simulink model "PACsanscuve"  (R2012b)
settings: Solver=ode3  StartTime=0.0  StopTime=50  RelTol=1e-3
libraries: simulink x1

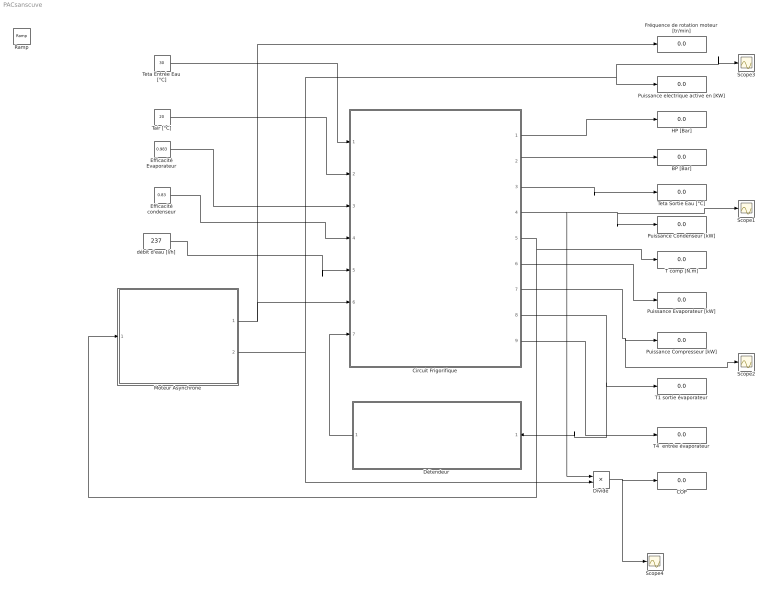
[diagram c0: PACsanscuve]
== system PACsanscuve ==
  BP [Bar] : Display
  COP : Display
  Circuit Frigorifique : Subsystem
  Divide : Product  Inputs=*/
  Détendeur : Subsystem
  Efficacité Evaporateur : Constant  Value=0.983
  Efficacité condenseur : Constant  Value=0.83
  Fréquence de rotation moteur [tr/min] : Display
  HP [Bar] : Display
  Moteur Asynchrone : Subsystem
  Puissance Compresseur [kW] : Display
  Puissance Condenseur [kW] : Display
  Puissance Evaporateur [kW] : Display
  Puissance electrique active en [KW] : Display
  Ramp : simulink/Sources/Ramp  slope=1  start=10  X0=30
  Scope{1..4} (4 alike) : Scope
  T comp [N.m] : Display
  T1 sortie évaporateur : Display
  T4  entrée évaporateur : Display
  Tair [°C] : Constant  Value=20
  Teta Entrée Eau [°C] : Constant  Value=30
  Teta Sortie Eau [°C] : Display
  débit d'eau [l/h] : Constant  Value=237
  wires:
  Efficacité Evaporateur/1 -> Circuit Frigorifique/3(Eff Evapo)
  débit d'eau [l/h]/1 -> Circuit Frigorifique/5(Qv eau [l/h])
  Circuit Frigorifique/1(HP [bar]) -> HP [Bar]/1
  Circuit Frigorifique/2(BP [bar]) -> BP [Bar]/1
  Circuit Frigorifique/3(Tse [°C]) -> Teta Sortie Eau [°C]/1
  Circuit Frigorifique/4(Pcond [kW]) -> Divide/1, Puissance Condenseur [kW]/1, Scope1/1
  Circuit Frigorifique/5(Tm [N.m]) -> Moteur Asynchrone/1(Tm [N.m]), T comp [N.m]/1
  Circuit Frigorifique/9(T4 [°C]) -> T4  entrée évaporateur/1
  Circuit Frigorifique/8(T1 [°C]) -> T1 sortie évaporateur/1, Détendeur/1(T1)
  Circuit Frigorifique/6(Pevapo [kW]) -> Puissance Evaporateur [kW]/1
  Divide/1 -> Scope4/1, COP/1
  Circuit Frigorifique/7(Pcomp [kW]) -> Scope2/1, Puissance Compresseur [kW]/1
  Efficacité condenseur/1 -> Circuit Frigorifique/4(effc)
  Détendeur/1(BP [Bar]) -> Circuit Frigorifique/7(BP[Bar])
  Moteur Asynchrone/2(Puissance Electrique active [W]) -> Scope3/1, Puissance electrique active en [KW]/1, Divide/2
  Moteur Asynchrone/1(N [tr/min]) -> Fréquence de rotation moteur [tr/min]/1, Circuit Frigorifique/6(N [tr/min])
  Tair [°C]/1 -> Circuit Frigorifique/2(Tair [°C])
  Teta Entrée Eau [°C]/1 -> Circuit Frigorifique/1(Tee [°C])

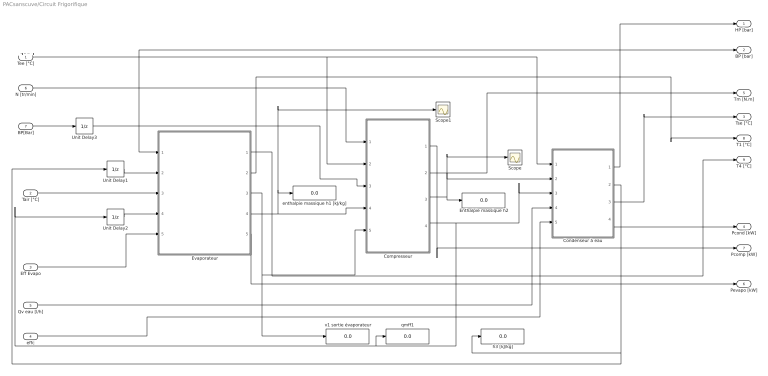
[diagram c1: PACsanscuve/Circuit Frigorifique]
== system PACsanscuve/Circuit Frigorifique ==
  note: +++++
  Tee [°C] : Inport
  Tair [°C] : Inport  Port=2
  Eff Evapo : Inport  Port=3
  effc : Inport  Port=4
  Qv eau [l/h] : Inport  Port=5
  N [tr/min] : Inport  Port=6
  BP[Bar] : Inport  Port=7
  Compresseur : Subsystem
  Condenseur à eau : Subsystem
  Enthalpie massique h2 : Display
  Evaporateur : Subsystem
  Scope : Scope
  Scope1 : Scope
  Unit Delay1 : UnitDelay  InitialCondition=300  SampleTime=-1
  Unit Delay2 : UnitDelay  InitialCondition=0.00001  SampleTime=-1
  Unit Delay3 : UnitDelay  InitialCondition=2.5  SampleTime=-1
  enthalpie massique h1 [kJ/kg] : Display
  h3 [kJ/kg] : Display
  qmff1 : Display
  v1 sortie évaporateur : Display
  HP [bar] : Outport
  BP [bar] : Outport  Port=2
  Tse [°C] : Outport  Port=3
  Pcond [kW] : Outport  Port=4
  Tm [N.m] : Outport  Port=5
  Pevapo [kW] : Outport  Port=6
  Pcomp [kW] : Outport  Port=7
  T1 [°C] : Outport  Port=8
  T4 [°C] : Outport  Port=9
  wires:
  Evaporateur/2(T1 [°C]) -> T1 [°C]/1
  N [tr/min]/1 -> Compresseur/1(N [tr/min])
  Evaporateur/5(Pévapo [kW]) -> Pevapo [kW]/1
  Tair [°C]/1 -> Evaporateur/3(Tair [°C])
  Condenseur à eau/3(Tse [°C]) -> Tse [°C]/1
  Unit Delay2/1 -> Evaporateur/4(qmff [kg/s])
  Condenseur à eau/1(HP [bar]) -> HP [bar]/1
  BP[Bar]/1 -> Unit Delay3/1
  Compresseur/4(qmff [kg/s]) -> Unit Delay2/1, qmff1/1, Condenseur à eau/3(qmff [kg/s])
  Tee [°C]/1 -> Compresseur/2(Tee [°C]), Condenseur à eau/1(Tee [°C])
  Eff Evapo/1 -> Evaporateur/5(Eff)
  Qv eau [l/h]/1 -> Condenseur à eau/4(qveau [l/h])
  Evaporateur/3(v1 [m3/kg]) -> v1 sortie évaporateur/1, Compresseur/5(v1 [m3/kg])
  Condenseur à eau/2(h3 [kJ/kg]) -> Unit Delay1/1, h3 [kJ/kg]/1
  Evaporateur/4(h1 [kJ/kg]) -> Compresseur/4(h1 [kJ/kg]), Scope1/1, enthalpie massique h1 [kJ/kg]/1
  Compresseur/3(h2 [kJ/kg]) -> Scope/1, Condenseur à eau/2(h2 [kJ/kg]), Enthalpie massique h2/1
  Compresseur/2(Tm [N.m]) -> Tm [N.m]/1
  Evaporateur/1(T4 [°C]) -> T4 [°C]/1
  Condenseur à eau/4(Pcond [kW]) -> Pcond [kW]/1
  Unit Delay1/1 -> Evaporateur/2(h3 [kJ/kg])
  Compresseur/1(Pcomp [kW]) -> Pcomp [kW]/1
  effc/1 -> Condenseur à eau/5(effc)
  Unit Delay3/1 -> BP [bar]/1, Compresseur/3(BP [bar]), Evaporateur/1(BP [bar])

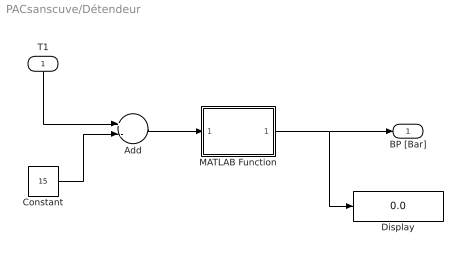
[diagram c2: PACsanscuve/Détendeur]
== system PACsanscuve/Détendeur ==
  T1 : Inport
  Add : Sum  Inputs=+-
  Constant : Constant  Value=15
  Display : Display
  MATLAB Function : MATLAB Function  TreatAsAtomicUnit=on
  BP [Bar] : Outport
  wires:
  Add/1 -> MATLAB Function/1(T)
  T1/1 -> Add/1
  MATLAB Function/1(BP) -> Display/1, BP [Bar]/1
  Constant/1 -> Add/2

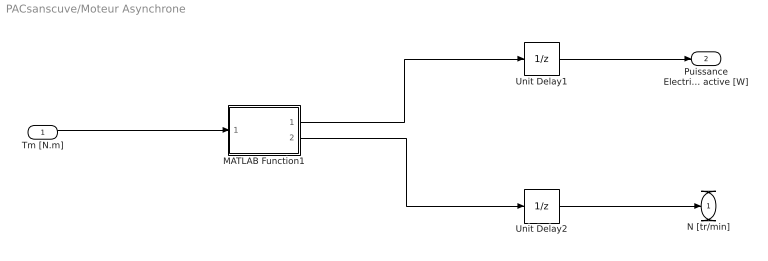
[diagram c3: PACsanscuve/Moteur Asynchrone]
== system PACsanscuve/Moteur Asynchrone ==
  Tm [N.m] : Inport
  MATLAB Function1 : MATLAB Function  TreatAsAtomicUnit=on
  Unit Delay1 : UnitDelay  InitialCondition=0.4  SampleTime=-1
  Unit Delay2 : UnitDelay  InitialCondition=1490  SampleTime=-1
  N [tr/min] : Outport
  Puissance Electrique active [W] : Outport  Port=2
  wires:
  Tm [N.m]/1 -> MATLAB Function1/1(Tm)
  MATLAB Function1/1(P) -> Unit Delay1/1
  MATLAB Function1/2(N) -> Unit Delay2/1
  Unit Delay1/1 -> Puissance Electrique active [W]/1
  Unit Delay2/1 -> N [tr/min]/1

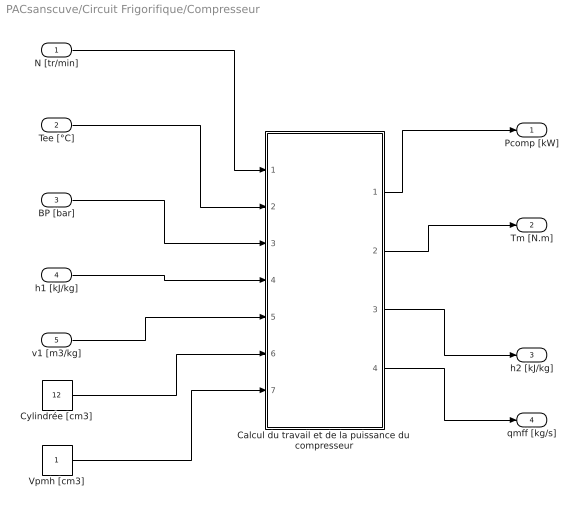
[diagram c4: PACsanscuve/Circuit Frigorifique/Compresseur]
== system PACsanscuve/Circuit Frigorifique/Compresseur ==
  N [tr/min] : Inport
  Tee [°C] : Inport  Port=2
  BP [bar] : Inport  Port=3
  h1 [kJ/kg] : Inport  Port=4
  v1 [m3/kg] : Inport  Port=5
  Calcul du travail et de la puissance du compresseur : MATLAB Function  TreatAsAtomicUnit=on
  Cylindrée [cm3] : Constant  Value=12
  Vpmh [cm3] : Constant
  Pcomp [kW] : Outport
  Tm [N.m] : Outport  Port=2
  h2 [kJ/kg] : Outport  Port=3
  qmff [kg/s] : Outport  Port=4
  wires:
  Calcul du travail et de la puissance du compresseur/4(qmff) -> qmff [kg/s]/1
  Calcul du travail et de la puissance du compresseur/2(Tm) -> Tm [N.m]/1
  h1 [kJ/kg]/1 -> Calcul du travail et de la puissance du compresseur/4(h1)
  Tee [°C]/1 -> Calcul du travail et de la puissance du compresseur/2(Tee)
  BP [bar]/1 -> Calcul du travail et de la puissance du compresseur/3(BP)
  Calcul du travail et de la puissance du compresseur/1(P) -> Pcomp [kW]/1
  Calcul du travail et de la puissance du compresseur/3(h2) -> h2 [kJ/kg]/1
  N [tr/min]/1 -> Calcul du travail et de la puissance du compresseur/1(N)
  v1 [m3/kg]/1 -> Calcul du travail et de la puissance du compresseur/5(v1)
  Cylindrée [cm3]/1 -> Calcul du travail et de la puissance du compresseur/6(cyl)
  Vpmh [cm3]/1 -> Calcul du travail et de la puissance du compresseur/7(Vpmh)

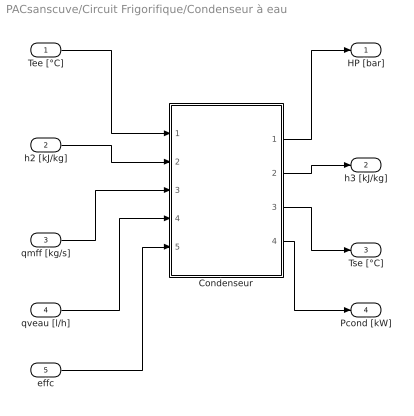
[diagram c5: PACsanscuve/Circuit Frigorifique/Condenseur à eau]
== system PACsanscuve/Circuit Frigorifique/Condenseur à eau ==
  Tee [°C] : Inport
  h2 [kJ/kg] : Inport  Port=2
  qmff [kg/s] : Inport  Port=3
  qveau [l/h] : Inport  Port=4
  effc : Inport  Port=5
  Condenseur : MATLAB Function  TreatAsAtomicUnit=on
  HP [bar] : Outport
  h3 [kJ/kg] : Outport  Port=2
  Tse [°C] : Outport  Port=3
  Pcond [kW] : Outport  Port=4
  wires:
  Tee [°C]/1 -> Condenseur/1(Tee)
  Condenseur/3(Tse) -> Tse [°C]/1
  Condenseur/1(HP) -> HP [bar]/1
  h2 [kJ/kg]/1 -> Condenseur/2(h2)
  qmff [kg/s]/1 -> Condenseur/3(qmff)
  qveau [l/h]/1 -> Condenseur/4(qveau)
  Condenseur/2(h3) -> h3 [kJ/kg]/1
  Condenseur/4(Pcond) -> Pcond [kW]/1
  effc/1 -> Condenseur/5(eff)

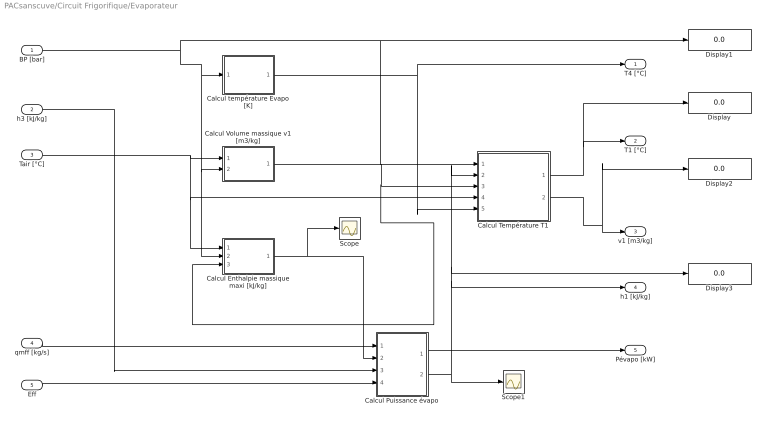
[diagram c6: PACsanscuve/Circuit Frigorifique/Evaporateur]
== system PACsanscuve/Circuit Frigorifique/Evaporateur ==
  BP [bar] : Inport
  h3 [kJ/kg] : Inport  Port=2
  Tair [°C] : Inport  Port=3
  qmff [kg/s] : Inport  Port=4
  Eff : Inport  Port=5
  Calcul Enthalpie massique maxi [kJ/kg] : MATLAB Function  TreatAsAtomicUnit=on
  Calcul Puissance évapo : MATLAB Function  TreatAsAtomicUnit=on
  Calcul Température T1 : MATLAB Function  TreatAsAtomicUnit=on
  Calcul Volume massique v1 [m3/kg] : MATLAB Function  TreatAsAtomicUnit=on
  Calcul température Evapo [K] : MATLAB Function  TreatAsAtomicUnit=on
  Display{,1..3} (4 alike) : Display
  Scope : Scope
  Scope1 : Scope
  T4 [°C] : Outport
  T1 [°C] : Outport  Port=2
  v1 [m3/kg] : Outport  Port=3
  h1 [kJ/kg] : Outport  Port=4
  Pévapo [kW] : Outport  Port=5
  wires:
  qmff [kg/s]/1 -> Calcul Puissance évapo/1(qmff)
  Calcul Enthalpie massique maxi [kJ/kg]/1(H) -> Scope/1, Calcul Puissance évapo/2(hmax)
  BP [bar]/1 -> Calcul Enthalpie massique maxi [kJ/kg]/2(P), Calcul Volume massique v1 [m3/kg]/2(P), Calcul température Evapo [K]/1(P), Display1/1, Calcul Température T1/1(P)
  Calcul température Evapo [K]/1(T) -> T4 [°C]/1, Calcul Température T1/5(T3)
  Tair [°C]/1 -> Calcul Enthalpie massique maxi [kJ/kg]/1(T), Calcul Température T1/4(T1max), Calcul Volume massique v1 [m3/kg]/1(T)
  Calcul Puissance évapo/1(Pevapo) -> Pévapo [kW]/1
  Eff/1 -> Calcul Puissance évapo/4(eff)
  Calcul Volume massique v1 [m3/kg]/1(v) -> Calcul Enthalpie massique maxi [kJ/kg]/3(v), Calcul Température T1/3(v)
  Calcul Température T1/2(v1) -> Display2/1, v1 [m3/kg]/1
  Calcul Température T1/1(T1) -> Display/1, T1 [°C]/1
  Calcul Puissance évapo/2(h1) -> h1 [kJ/kg]/1, Display3/1, Calcul Température T1/2(h), Scope1/1
  h3 [kJ/kg]/1 -> Calcul Puissance évapo/3(h3)
